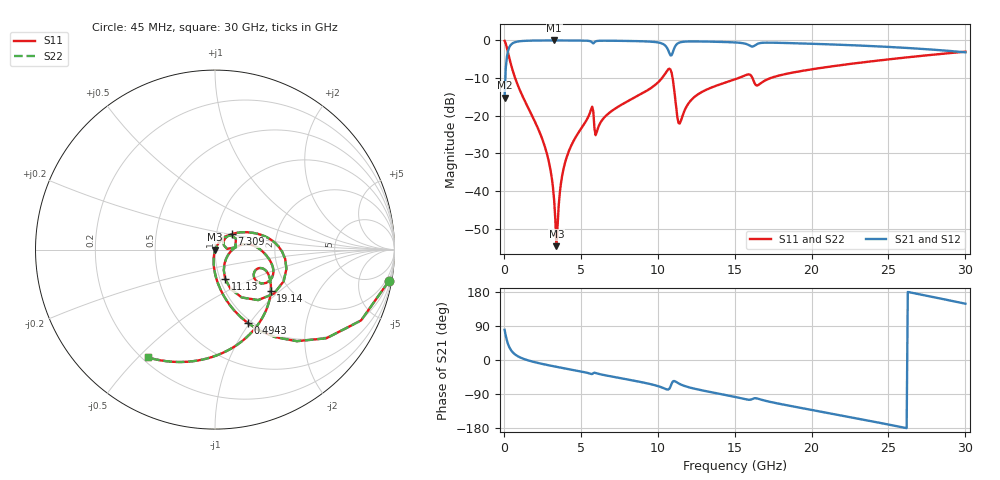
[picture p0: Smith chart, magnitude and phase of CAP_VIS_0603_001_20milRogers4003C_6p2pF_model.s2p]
! S-parameter model data by Modelithics Inc.  support@modelithics.com  813-866-6335  Tampa FL USA
! S-Parameter data specifications:
! Substrate: 20-mil Rogers 4003C, substrate thickness, H=0.508mm, Dielectric constant, Er=3.75
! PCB Mounting Pad Footprint: Pad width, PadW=0.90mm , Pad length, PadL=1.00mm , Pad gap, PadG (edge-to-edge)=1.00mm , Reference planes=3.0mm apart
! Created Wed Nov 18 13:24:10 2015
# hz S ma R 50
! 2 Port Network Data from SP1.SP block
! freq  magS11  angS11  magS21  angS21  magS12  angS12  magS22  angS22
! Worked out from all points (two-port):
!   401 points, 45 MHz to 30 GHz, reference 50 ohm
!   highest |S21| = -0.02 dB at 3.265 GHz (marker M1); lowest = -15.2 dB at 45 MHz (marker M2)
!   |S21| within 3 dB of the highest: 256.8 MHz to 10.72 GHz (10.46 GHz wide, 191 % of centre); 10.99 GHz to 29.59 GHz (18.6 GHz wide, 91.7 % of centre)
!   lowest |S11| = -54.7 dB at 3.415 GHz (marker M3), VSWR 1.00, Z = 50.2 - j0.0966 ohm
!   |S11| at or under -10 dB: 730.6 MHz to 10.28 GHz (9.548 GHz wide, 173 % of centre); 10.97 GHz to 15.25 GHz (4.283 GHz wide, 32.7 % of centre); 16.16 GHz to 17.34 GHz (1.182 GHz wide, 7.06 % of centre)
!   |S22| runs from -54.7 to -0.1 dB; largest |S21 - S12| = 0
!   S11 on the Smith chart (normalised r, x): 45 MHz: 1, -11; 494.3 MHz: 0.96, -0.99; 7.309 GHz: 1.19, +0.21; 11.13 GHz: 1.06, -0.36; 19.14 GHz: 1.62, -0.87; 30 GHz: 0.22, -0.53
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4.5e7  0.9847 -10.3  0.174 79.7  0.174 79.7  0.9847 -10.3
2.696625e8  0.6844 -48.2  0.7287 41.8  0.7287 41.8  0.6844 -48.2
4.94325e8  0.4506 -65.8  0.8921 24.2  0.8921 24.2  0.4506 -65.8
2.666062e9  0.03854 -99.6  0.9975 -11.9  0.9975 -11.9  0.03854 -99.6
3.0405e9  0.01838 -99.8  0.9979 -15.0  0.9979 -15.0  0.01838 -99.8
3.265162e9  0.007564 -93.4  0.9979 -16.8  0.9979 -16.8  0.007564 -93.4
3.414938e9  0.001851 -31.4  0.9979 -18.0  0.9979 -18.0  0.001851 -31.4
4.014038e9  0.02539 62.8  0.9973 -22.7  0.9973 -22.7  0.02539 62.8
5.062462e9  0.06949 56.6  0.9939 -30.7  0.9939 -30.7  0.06949 56.6
5.661562e9  0.1205 40.3  0.9654 -36.6  0.9654 -36.6  0.1205 40.3
6.036e9  0.06061 38.8  0.9811 -35.2  0.9811 -35.2  0.06061 38.8
7.309088e9  0.1271 42.4  0.9875 -45.9  0.9875 -45.9  0.1271 42.4
1.007992e10  0.2845 15.4  0.9338 -69.7  0.9338 -69.7  0.2845 15.4
1.075391e10  0.4214 -24.8  0.6794 -76.0  0.6794 -76.0  0.4214 -24.8
1.112835e10  0.1725 -70.8  0.8311 -56.3  0.8311 -56.3  0.1725 -70.8
1.14279e10  0.07869 -22.4  0.9382 -63.3  0.9382 -63.3  0.07869 -22.4
1.247632e10  0.1834 9.3  0.9688 -76.5  0.9688 -76.5  0.1834 9.3
1.50225e10  0.3042 -9.7  0.9393 -97.4  0.9393 -97.4  0.3042 -9.7
1.914131e10  0.3858 -36.2  0.9134 -125.2  0.9134 -125.2  0.3858 -36.2
2.003996e10  0.4138 -42.9  0.9016 -132.0  0.9016 -132.0  0.4138 -42.9
2.505742e10  0.5613 -81.4  0.8181 -170.8  0.8181 -170.8  0.5613 -81.4
3e10  0.7081 -122.0  0.6942 148.5  0.6942 148.5  0.7081 -122.0
